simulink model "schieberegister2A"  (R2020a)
settings: Solver=VariableStepDiscrete  StartTime=0.0  StopTime=Inf  RelTol=1e-3  EnableMultiTasking=on

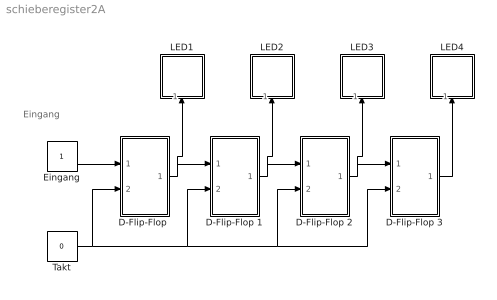
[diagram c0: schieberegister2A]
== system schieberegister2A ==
  note: Eingang
  "D-Flip-Flop " : Subsystem  mask(DFlipFlop){s0=off}
      mask prompts: s0 "Initially on"
      mask help: D Flip-Flop Block
  D-Flip-Flop 1 : Subsystem  mask(DFlipFlop){s0=off}
      mask prompts: s0 "Initially on"
      mask help: D Flip-Flop Block
  D-Flip-Flop 2 : Subsystem  mask(DFlipFlop){s0=off}
      mask prompts: s0 "Initially on"
      mask help: D Flip-Flop Block
  D-Flip-Flop 3 : Subsystem  mask(DFlipFlop){s0=off}
      mask prompts: s0 "Initially on"
      mask help: D Flip-Flop Block
  Eingang : Constant  OutDataTypeStr=double
  LED1 : Subsystem  mask(LED){on_color=[0.0, 1.0, 0.0], off_color=[0.0, 0.2, 0.0]}
      mask prompts: on_color "Color for "on" state"; off_color "Color for "off" state"
      mask help: Display of a binary signal
  LED2 : Subsystem  mask(LED){on_color=[0.0, 1.0, 0.0], off_color=[0.0, 0.2, 0.0]}
      mask prompts: on_color "Color for "on" state"; off_color "Color for "off" state"
      mask help: Display of a binary signal
  LED3 : Subsystem  mask(LED){on_color=[0.0, 1.0, 0.0], off_color=[0.0, 0.2, 0.0]}
      mask prompts: on_color "Color for "on" state"; off_color "Color for "off" state"
      mask help: Display of a binary signal
  LED4 : Subsystem  mask(LED){on_color=[0.0, 1.0, 0.0], off_color=[0.0, 0.2, 0.0]}
      mask prompts: on_color "Color for "on" state"; off_color "Color for "off" state"
      mask help: Display of a binary signal
  Takt : Constant  Value=0  OutDataTypeStr=double
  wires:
  "D-Flip-Flop "/1(Q) -> D-Flip-Flop 1/1(D), LED1/1(In)
  D-Flip-Flop 1/1(Q) -> D-Flip-Flop 2/1(D), LED2/1(In)
  D-Flip-Flop 2/1(Q) -> D-Flip-Flop 3/1(D), LED3/1(In)
  Eingang/1 -> "D-Flip-Flop "/1(D)
  Takt/1 -> "D-Flip-Flop "/2(CLK), D-Flip-Flop 1/2(CLK), D-Flip-Flop 2/2(CLK), D-Flip-Flop 3/2(CLK)
  D-Flip-Flop 3/1(Q) -> LED4/1(In)

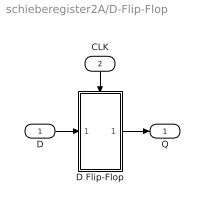
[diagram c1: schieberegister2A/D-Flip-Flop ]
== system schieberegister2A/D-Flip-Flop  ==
  D : Inport
  CLK : Inport  Port=2
  D Flip-Flop : Subsystem  TreatAsAtomicUnit=on
  Q : Outport  InitialOutput=0
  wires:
  CLK/1 -> D Flip-Flop/Trigger
  D Flip-Flop/1(Q) -> Q/1
  D/1 -> D Flip-Flop/1(D)

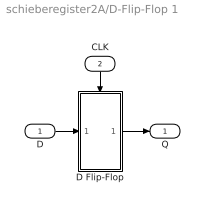
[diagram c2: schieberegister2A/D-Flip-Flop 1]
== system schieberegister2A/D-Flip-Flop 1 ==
  D : Inport
  CLK : Inport  Port=2
  D Flip-Flop : Subsystem  TreatAsAtomicUnit=on
  Q : Outport  InitialOutput=0
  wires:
  D/1 -> D Flip-Flop/1(D)
  D Flip-Flop/1(Q) -> Q/1
  CLK/1 -> D Flip-Flop/Trigger

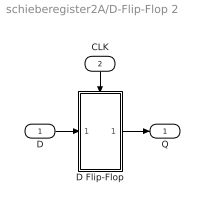
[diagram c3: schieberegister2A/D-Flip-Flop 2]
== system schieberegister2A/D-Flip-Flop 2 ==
  D : Inport
  CLK : Inport  Port=2
  D Flip-Flop : Subsystem  TreatAsAtomicUnit=on
  Q : Outport  InitialOutput=0
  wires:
  CLK/1 -> D Flip-Flop/Trigger
  D Flip-Flop/1(Q) -> Q/1
  D/1 -> D Flip-Flop/1(D)

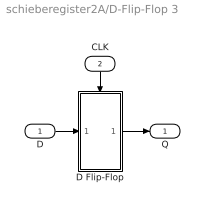
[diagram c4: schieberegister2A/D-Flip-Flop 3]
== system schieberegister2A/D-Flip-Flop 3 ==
  D : Inport
  CLK : Inport  Port=2
  D Flip-Flop : Subsystem  TreatAsAtomicUnit=on
  Q : Outport  InitialOutput=0
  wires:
  D/1 -> D Flip-Flop/1(D)
  D Flip-Flop/1(Q) -> Q/1
  CLK/1 -> D Flip-Flop/Trigger

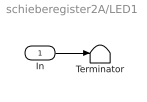
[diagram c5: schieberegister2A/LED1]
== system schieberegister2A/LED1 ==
  In : Inport
  Terminator : Terminator
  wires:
  In/1 -> Terminator/1

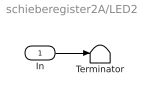
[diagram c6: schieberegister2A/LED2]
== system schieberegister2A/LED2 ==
  In : Inport
  Terminator : Terminator
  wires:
  In/1 -> Terminator/1

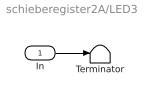
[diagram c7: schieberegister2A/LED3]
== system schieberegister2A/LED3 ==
  In : Inport
  Terminator : Terminator
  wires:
  In/1 -> Terminator/1

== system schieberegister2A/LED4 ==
  In : Inport
  Terminator : Terminator
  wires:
  In/1 -> Terminator/1

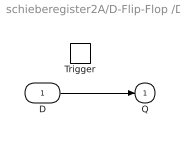
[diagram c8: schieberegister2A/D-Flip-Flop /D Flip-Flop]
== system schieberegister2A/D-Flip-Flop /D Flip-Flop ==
  D : Inport
  Trigger : TriggerPort  TriggerType=falling  VariantControl=Variant
  Q : Outport  InitialOutput=s0
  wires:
  D/1 -> Q/1

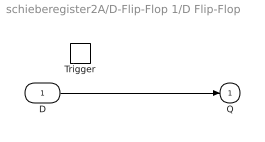
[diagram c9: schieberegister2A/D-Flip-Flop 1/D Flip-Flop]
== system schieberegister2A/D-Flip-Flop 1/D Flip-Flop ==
  D : Inport
  Trigger : TriggerPort  TriggerType=falling  VariantControl=Variant
  Q : Outport  InitialOutput=s0
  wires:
  D/1 -> Q/1

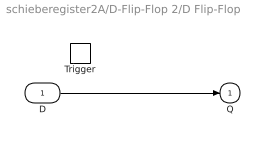
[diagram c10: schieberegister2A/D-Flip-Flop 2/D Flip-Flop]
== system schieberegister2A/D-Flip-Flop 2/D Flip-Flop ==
  D : Inport
  Trigger : TriggerPort  TriggerType=falling  VariantControl=Variant
  Q : Outport  InitialOutput=s0
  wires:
  D/1 -> Q/1

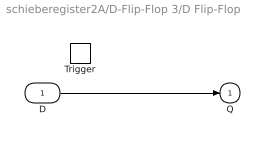
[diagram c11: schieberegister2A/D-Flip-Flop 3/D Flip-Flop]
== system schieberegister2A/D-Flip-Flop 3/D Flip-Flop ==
  D : Inport
  Trigger : TriggerPort  TriggerType=falling  VariantControl=Variant
  Q : Outport  InitialOutput=s0
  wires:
  D/1 -> Q/1
